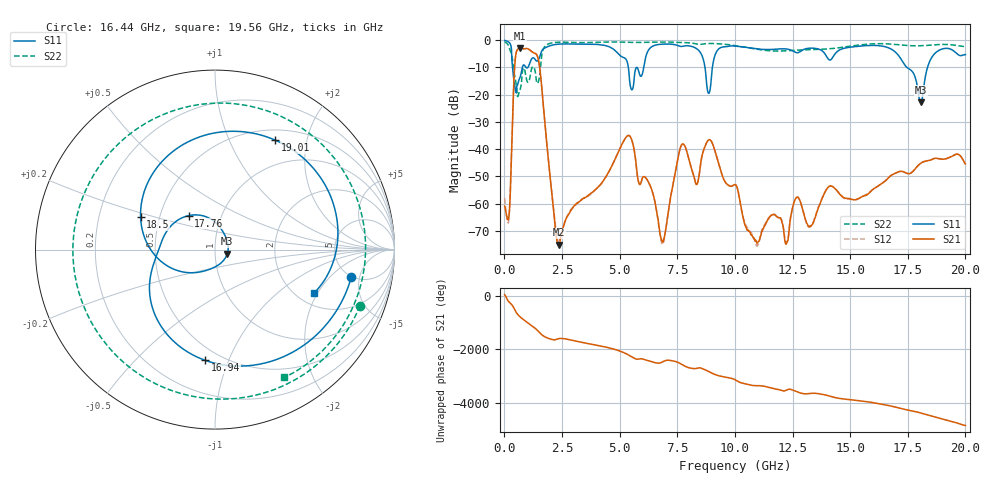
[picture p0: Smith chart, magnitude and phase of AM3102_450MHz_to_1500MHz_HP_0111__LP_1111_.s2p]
!Agilent Technologies,E8364B,MY43040894,A.07.50.67
!Agilent E8364B: A.07.50.67
!Date: Thursday, January 11, 2018 05:55:13
!Correction: S11(Full 2 Port(1,2))
!S21(Full 2 Port(1,2))
!S12(Full 2 Port(1,2))
!S22(Full 2 Port(1,2))
!S2P File: Measurements: S11, S21, S12, S22:
# Hz S  dB  R 50
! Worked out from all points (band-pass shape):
!   1601 points, 10 MHz to 20 GHz, reference 50 ohm
!   highest |S21| = -2.94 dB at 684.7 MHz (marker M1); lowest = -75.2 dB at 2.359 GHz (marker M2)
!   |S21| within 3 dB of the highest: 484 MHz to 1.438 GHz (953.9 MHz wide, 99.3 % of centre)
!   lowest |S11| = -22.8 dB at 18.06 GHz (marker M3), VSWR 1.16, Z = 57.3 - j2.57 ohm
!   |S11| at or under -10 dB: 356 MHz to 779.4 MHz (423.4 MHz wide, 74.6 % of centre); 5.379 GHz to 5.731 GHz (351.5 MHz wide, 6.33 % of centre); 17.47 GHz to 18.36 GHz (889.2 MHz wide, 4.96 % of centre)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
!   |S22| runs from -20.7 to -0.5 dB; largest |S21 - S12| = 0.0016
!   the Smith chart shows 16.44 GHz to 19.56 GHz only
!   S11 on the Smith chart (normalised r, x): 16.44 GHz: 4.91, -3.77; 16.94 GHz: 0.41, -0.83; 17.76 GHz: 0.70, +0.28; 18.5 GHz: 0.39, +0.18; 19.01 GHz: 0.63, +1.50; 19.56 GHz: 2.47, -1.87
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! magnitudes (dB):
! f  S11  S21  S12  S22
! 10 MHz  -0.1  -60.9  -58.0  -0.5
! 184.9 MHz  -0.6  -65.5  -66.3  -2.1
! 459.8 MHz  -17.4  -8.0  -8.0  -13.6
! 684.7 MHz  -13.5  -2.9  -2.9  -18.0
! 1.484 GHz  -7.0  -7.5  -7.5  -15.0
! 2.359 GHz  -1.4  -75.2  -74.4  -0.7
! 3.346 GHz  -1.4  -58.6  -58.4  -0.9
! 5.395 GHz  -11.0  -35.0  -35.0  -0.7
! 6.682 GHz  -1.6  -66.7  -67.0  -0.7
! 7.731 GHz  -2.2  -38.1  -38.1  -0.8
! 10.01 GHz  -2.1  -53.0  -53.0  -2.0
! 10.95 GHz  -3.2  -74.6  -75.6  -3.3
! 13.34 GHz  -2.9  -67.9  -67.8  -3.4
! 16.44 GHz  -2.2  -52.2  -52.2  -1.3
! 16.68 GHz  -2.8  -50.4  -50.4  -1.3
! 16.94 GHz  -4.2  -49.0  -48.9  -1.5
! 17.76 GHz  -12.4  -47.8  -47.8  -2.0
! 18.06 GHz  -22.8  -45.2  -45.2  -2.0
! 18.5 GHz  -6.9  -44.0  -44.0  -1.8
! 19.01 GHz  -3.2  -43.7  -43.7  -1.5
! 19.56 GHz  -4.4  -42.0  -42.0  -1.8
! 20 GHz  -5.2  -45.5  -45.5  -2.3
